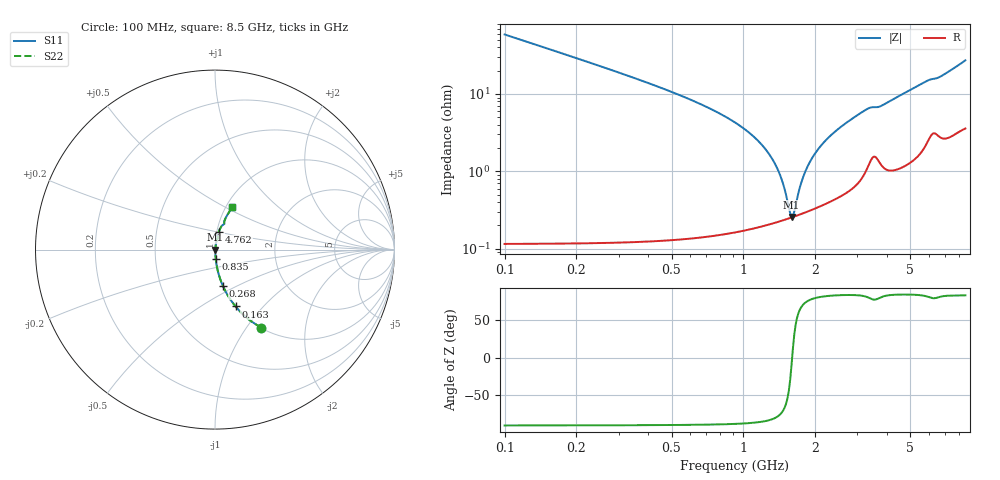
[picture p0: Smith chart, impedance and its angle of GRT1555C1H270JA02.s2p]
!Murata Part Number: GRT1555C1H270JA02
!These Parameters are Measured in Series Mode Connection
!Data Generated on Jun 19, 2026
!  o--ll--o
!Port1  Port2
!  o------o
!Operation Temp=25[degC], DC Bias Voltage=0[V]
!Freq. Start=100[MHz] Stop=9[GHz] 401[Steps]
# Hz S RI R 50
!Freq.(Hz) S11(Real) S11(Imag) S21(Real) S21(Imag) S12(Real) S12(Imag) S22(Real) S22(Imag)
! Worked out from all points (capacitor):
!   401 points, 100 MHz to 8.5 GHz, reference 50 ohm
!   read as one part in series: C = 27 pF near 142 MHz
!   lowest |Z| = 257 mohm at 1.591 GHz (marker M1)
!   series resonance near 1.6 GHz, so ESL is about 370 pH
!   S11 on the Smith chart (normalised r, x): 100 MHz: 1.00, -1.17; 163 MHz: 1.00, -0.72; 268 MHz: 1.00, -0.43; 835 MHz: 1.00, -0.10; 4.762 GHz: 1.02, +0.21; 8.5 GHz: 1.07, +0.54
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1e8  0.2568 -0.4359  0.7432 0.4359  0.7432 0.4359  0.2568 -0.4359
1.63e8  0.1144 -0.3166  0.8856 0.3166  0.8856 0.3166  0.1144 -0.3166
2.68e8  0.0448 -0.204  0.9552 0.204  0.9552 0.204  0.0448 -0.204
4.78e8  0.0137 -0.1107  0.9863 0.1107  0.9863 0.1107  0.0137 -0.1107
8.35e8  0.00417 -0.0512  0.9958 0.0512  0.9958 0.0512  0.00417 -0.0512
1.276e9  0.00233 -0.0168  0.9977 0.0168  0.9977 0.0168  0.00233 -0.0168
1.402e9  0.00233 -0.00977  0.9977 0.00977  0.9977 0.00977  0.00233 -0.00977
1.507e9  0.00241 -0.00441  0.9976 0.00441  0.9976 0.00441  0.00241 -0.00441
1.549e9  0.00247 -0.00238  0.9975 0.00238  0.9975 0.00238  0.00247 -0.00238
1.591e9  0.00253 -0.000394  0.9975 0.000394  0.9975 0.000394  0.00253 -0.000394
1.633e9  0.00261 0.00154  0.9974 -0.00154  0.9974 -0.00154  0.00261 0.00154
1.717e9  0.00278 0.00527  0.9972 -0.00527  0.9972 -0.00527  0.00278 0.00527
1.801e9  0.00299 0.00884  0.997 -0.00884  0.997 -0.00884  0.00299 0.00884
2.011e9  0.00363 0.0172  0.9964 -0.0172  0.9964 -0.0172  0.00363 0.0172
2.368e9  0.00511 0.0303  0.9949 -0.0303  0.9949 -0.0303  0.00511 0.0303
2.914e9  0.00868 0.049  0.9913 -0.049  0.9913 -0.049  0.00868 0.049
3.334e9  0.0156 0.0623  0.9844 -0.0623  0.9844 -0.0623  0.0156 0.0623
4.3e9  0.0176 0.0848  0.9824 -0.0848  0.9824 -0.0848  0.0176 0.0848
4.762e9  0.0219 0.0999  0.9781 -0.0999  0.9781 -0.0999  0.0219 0.0999
5.707e9  0.0376 0.1318  0.9624 -0.1318  0.9624 -0.1318  0.0376 0.1318
7.114e9  0.0572 0.1714  0.9428 -0.1714  0.9428 -0.1714  0.0572 0.1714
8.5e9  0.0961 0.2358  0.9039 -0.2358  0.9039 -0.2358  0.0961 0.2358
